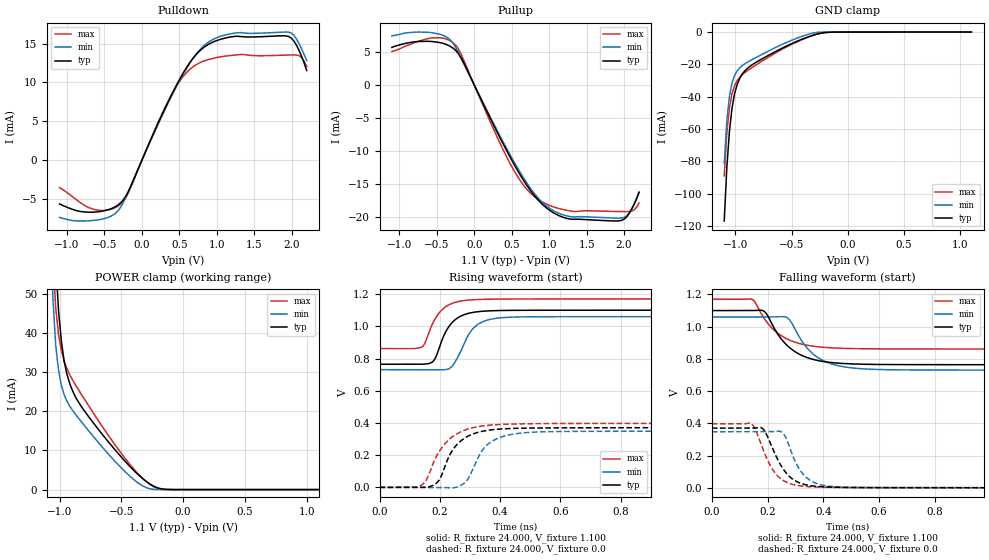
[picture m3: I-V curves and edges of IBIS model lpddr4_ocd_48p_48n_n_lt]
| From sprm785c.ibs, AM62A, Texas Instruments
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|   Model lpddr4_ocd_48p_48n_n_lt
[Model] lpddr4_ocd_48p_48n_n_lt
Model_type I/O
Polarity   Non-Inverting
Enable   Active-High
Vinl =  0.113V
Vinh =  0.253V
Vmeas =  0.183V
C_comp   2.242pF   2.051pF   2.315pF
[Model Spec]
Vinh   0.253V   0.247V   0.265V
Vinl   0.113V   0.107V   0.125V
Vmeas   0.183V   0.176V   0.195V
[Temperature Range]   25.000   -40.000   -40.000
[Voltage Range]   1.100V   1.060V   1.170V
[Pullup Reference]   1.100V   1.060V   1.170V
[Pulldown Reference]   0.0V   0.0V   0.0V
[C Comp Corner]
C_comp   2.242pF   2.051pF   2.315pF
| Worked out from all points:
|   slope of the pulldown table from 0 to 0.165 V, typ, clamps not added: 45.1 ohm
|   slope of the pullup table from 0 to 0.165 V, typ, clamps not added: 42.1 ohm
|   GND clamp passes 1 mA (typ) near -0.26 V on its own axis
|   POWER clamp passes 1 mA (typ) near -0.24 V on its own axis
|   rising waveform, R_fixture 24.000, V_fixture 1.100: 20-80 % time 54.5ps typ, 58.6ps min, 54.3ps max; typ from 0.764 V to 1.1 V
|   rising waveform, R_fixture 24.000, V_fixture 0.0: 20-80 % time 69.5ps typ, 69.4ps min, 80.8ps max; typ from 0.001 V to 0.371 V
|   falling waveform, R_fixture 24.000, V_fixture 1.100: 20-80 % time 101ps typ, 96.1ps min, 102ps max; typ from 1.1 V to 0.764 V
|   falling waveform, R_fixture 24.000, V_fixture 0.0: 20-80 % time 70.8ps typ, 62.5ps min, 66.2ps max; typ from 0.371 V to 0.001 V
[Pulldown]
|Voltage   I(typ)   I(min)   I(max)
-1.1V     -5.643mA   -7.369mA   -3.548mA
-658mV    -6.702mA   -7.776mA   -6.297mA
-284mV    -5.484mA   -6.063mA   -5.663mA
-181mV    -4.033mA   -4.01mA    -4.194mA
227mV     4.993mA    4.851mA    5.074mA
465mV     9.726mA    9.54mA     9.569mA
703mV     13.36mA    13.37mA    12.15mA
907mV     15mA       15.3mA     13mA
1.281V    15.93mA    16.39mA    13.56mA
1.962V    15.89mA    16.46mA    13.52mA
2.098V    14.11mA    14.97mA    13.44mA
2.2V      11.53mA    12.81mA    12.03mA
[Pullup]
|Voltage   I(typ)   I(min)   I(max)
-1.1V     5.717mA    7.477mA    5.093mA
-556mV    6.609mA    7.943mA    7.174mA
-386mV    6.227mA    7.4mA      7.045mA
-249mV    5.279mA    5.734mA    6.068mA
329mV     -7.689mA   -7.412mA   -8.482mA
567mV     -12.77mA   -12.4mA    -13.71mA
771mV     -16.35mA   -16.02mA   -16.65mA
1.043V    -19.32mA   -19.01mA   -18.47mA
1.281V    -20.38mA   -20.01mA   -19.14mA
1.962V    -20.59mA   -20.23mA   -19.23mA
2.064V    -19.58mA   -19.5mA    -19.24mA
2.2V      -16.36mA   -16.2mA    -17.91mA
[GND_clamp]
|Voltage   I(typ)   I(min)   I(max)
-1.1V     -116.8mA   -81.18mA   -88.94mA
-1.077V   -83.96mA   -55.01mA   -62.39mA
-1.054V   -61.6mA    -39.81mA   -46.82mA
-1.031V   -47.19mA   -31.46mA   -38.11mA
-1.008V   -38.16mA   -26.8mA    -33.12mA
-985mV    -32.43mA   -23.99mA   -30.04mA
-962mV    -28.65mA   -22.13mA   -27.95mA
-917mV    -24.03mA   -19.66mA   -25.07mA
-871mV    -21.2mA    -17.79mA   -22.81mA
-481mV    -6.583mA   -4.567mA   -6.994mA
-229mV    -598.7uA   -45.01uA   -573.1uA
1.1V      0A         0A         0A
[POWER_clamp]
|Voltage   I(typ)   I(min)   I(max)
-1.1V     158.5mA    112mA      122.8mA
-1.054V   78.43mA    48.87mA    58.82mA
-1.031V   58.13mA    36.84mA    46.37mA
-1.008V   45.61mA    30.38mA    39.54mA
-985mV    37.81mA    26.62mA    35.43mA
-940mV    29.44mA    22.56mA    30.8mA
-894mV    25.17mA    20.2mA     27.97mA
-825mV    21.26mA    17.35mA    24.37mA
-367mV    3.904mA    1.752mA    4.09mA
-252mV    1.127mA    118.9uA    960.8uA
-160mV    128.1uA    2.957uA    54.28uA
1.1V      0A         0A         0A
[Ramp]
| variable   typ   min   max
dV/dt_r   0.222/69.366p   0.210/69.521p   0.238/80.817p
dV/dt_f   0.201/0.101n   0.197/96.083p   0.185/0.102n
R_load = 24.000
[Rising Waveform]
R_fixture= 24.000
V_fixture= 1.100
V_fixture_min= 1.060
V_fixture_max= 1.170
|time   V(typ)   V(min)   V(max)
0s        764.4mV    730.8mV    861.7mV
139ps     763.9mV    730.8mV    870.3mV
150ps     765.3mV    730.8mV    893.5mV
172ps     774.7mV    730.8mV    999.8mV
198ps     865.8mV    730.2mV    1.083V
230ps     997.9mV    736.2mV    1.133V
251ps     1.041V     779.9mV    1.148V
308ps     1.085V     981.2mV    1.164V
373ps     1.096V     1.045V     1.168V
5ns       1.1V       1.06V      1.17V
[Rising Waveform]
R_fixture= 24.000
V_fixture= 0.0
V_fixture_min= 0.0
V_fixture_max= 0.0
|time   V(typ)   V(min)   V(max)
0s        670.9uV    48.03uV    1.426mV
133ps     616.1uV    47.21uV    7.237mV
156ps     1.296mV    48.71uV    49.1mV
179ps     15.01mV    45.33uV    154.3mV
215ps     120.9mV    -122.8uV   267.2mV
262ps     276.2mV    6.418mV    338.6mV
292ps     317mV      49.37mV    361.9mV
349ps     351.6mV    249.8mV    383.3mV
412ps     364mV      317.9mV    391.8mV
5ns       371.2mV    350.8mV    397.9mV
[Falling Waveform]
R_fixture= 24.000
V_fixture= 1.100
V_fixture_min= 1.060
V_fixture_max= 1.170
|time   V(typ)   V(min)   V(max)
0s        1.1V       1.06V      1.17V
143ps     1.1V       1.06V      1.171V
185ps     1.098V     1.06V      1.059V
222ps     995.8mV    1.06V      981mV
266ps     890.8mV    1.059V     927.3mV
284ps     863mV      1.03V      913mV
332ps     814.9mV    888.8mV    888.4mV
369ps     794.6mV    822.8mV    877.8mV
498ps     769.4mV    745.2mV    864.5mV
5ns       764.4mV    730.8mV    861.7mV
[Falling Waveform]
R_fixture= 24.000
V_fixture= 0.0
V_fixture_min= 0.0
V_fixture_max= 0.0
|time   V(typ)   V(min)   V(max)
0s        370.7mV    348.4mV    397.5mV
143ps     370.5mV    348.4mV    397.9mV
186ps     361.3mV    348.4mV    228.8mV
216ps     252.6mV    348.3mV    119.9mV
249ps     135.9mV    347.8mV    54.6mV
265ps     95.88mV    312.7mV    37.4mV
314ps     31.48mV    116.8mV    12.9mV
362ps     11.65mV    37.55mV    5.759mV
585ps     1.504mV    1.098mV    1.913mV
5ns       670.5uV    47.95uV    1.427mV
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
